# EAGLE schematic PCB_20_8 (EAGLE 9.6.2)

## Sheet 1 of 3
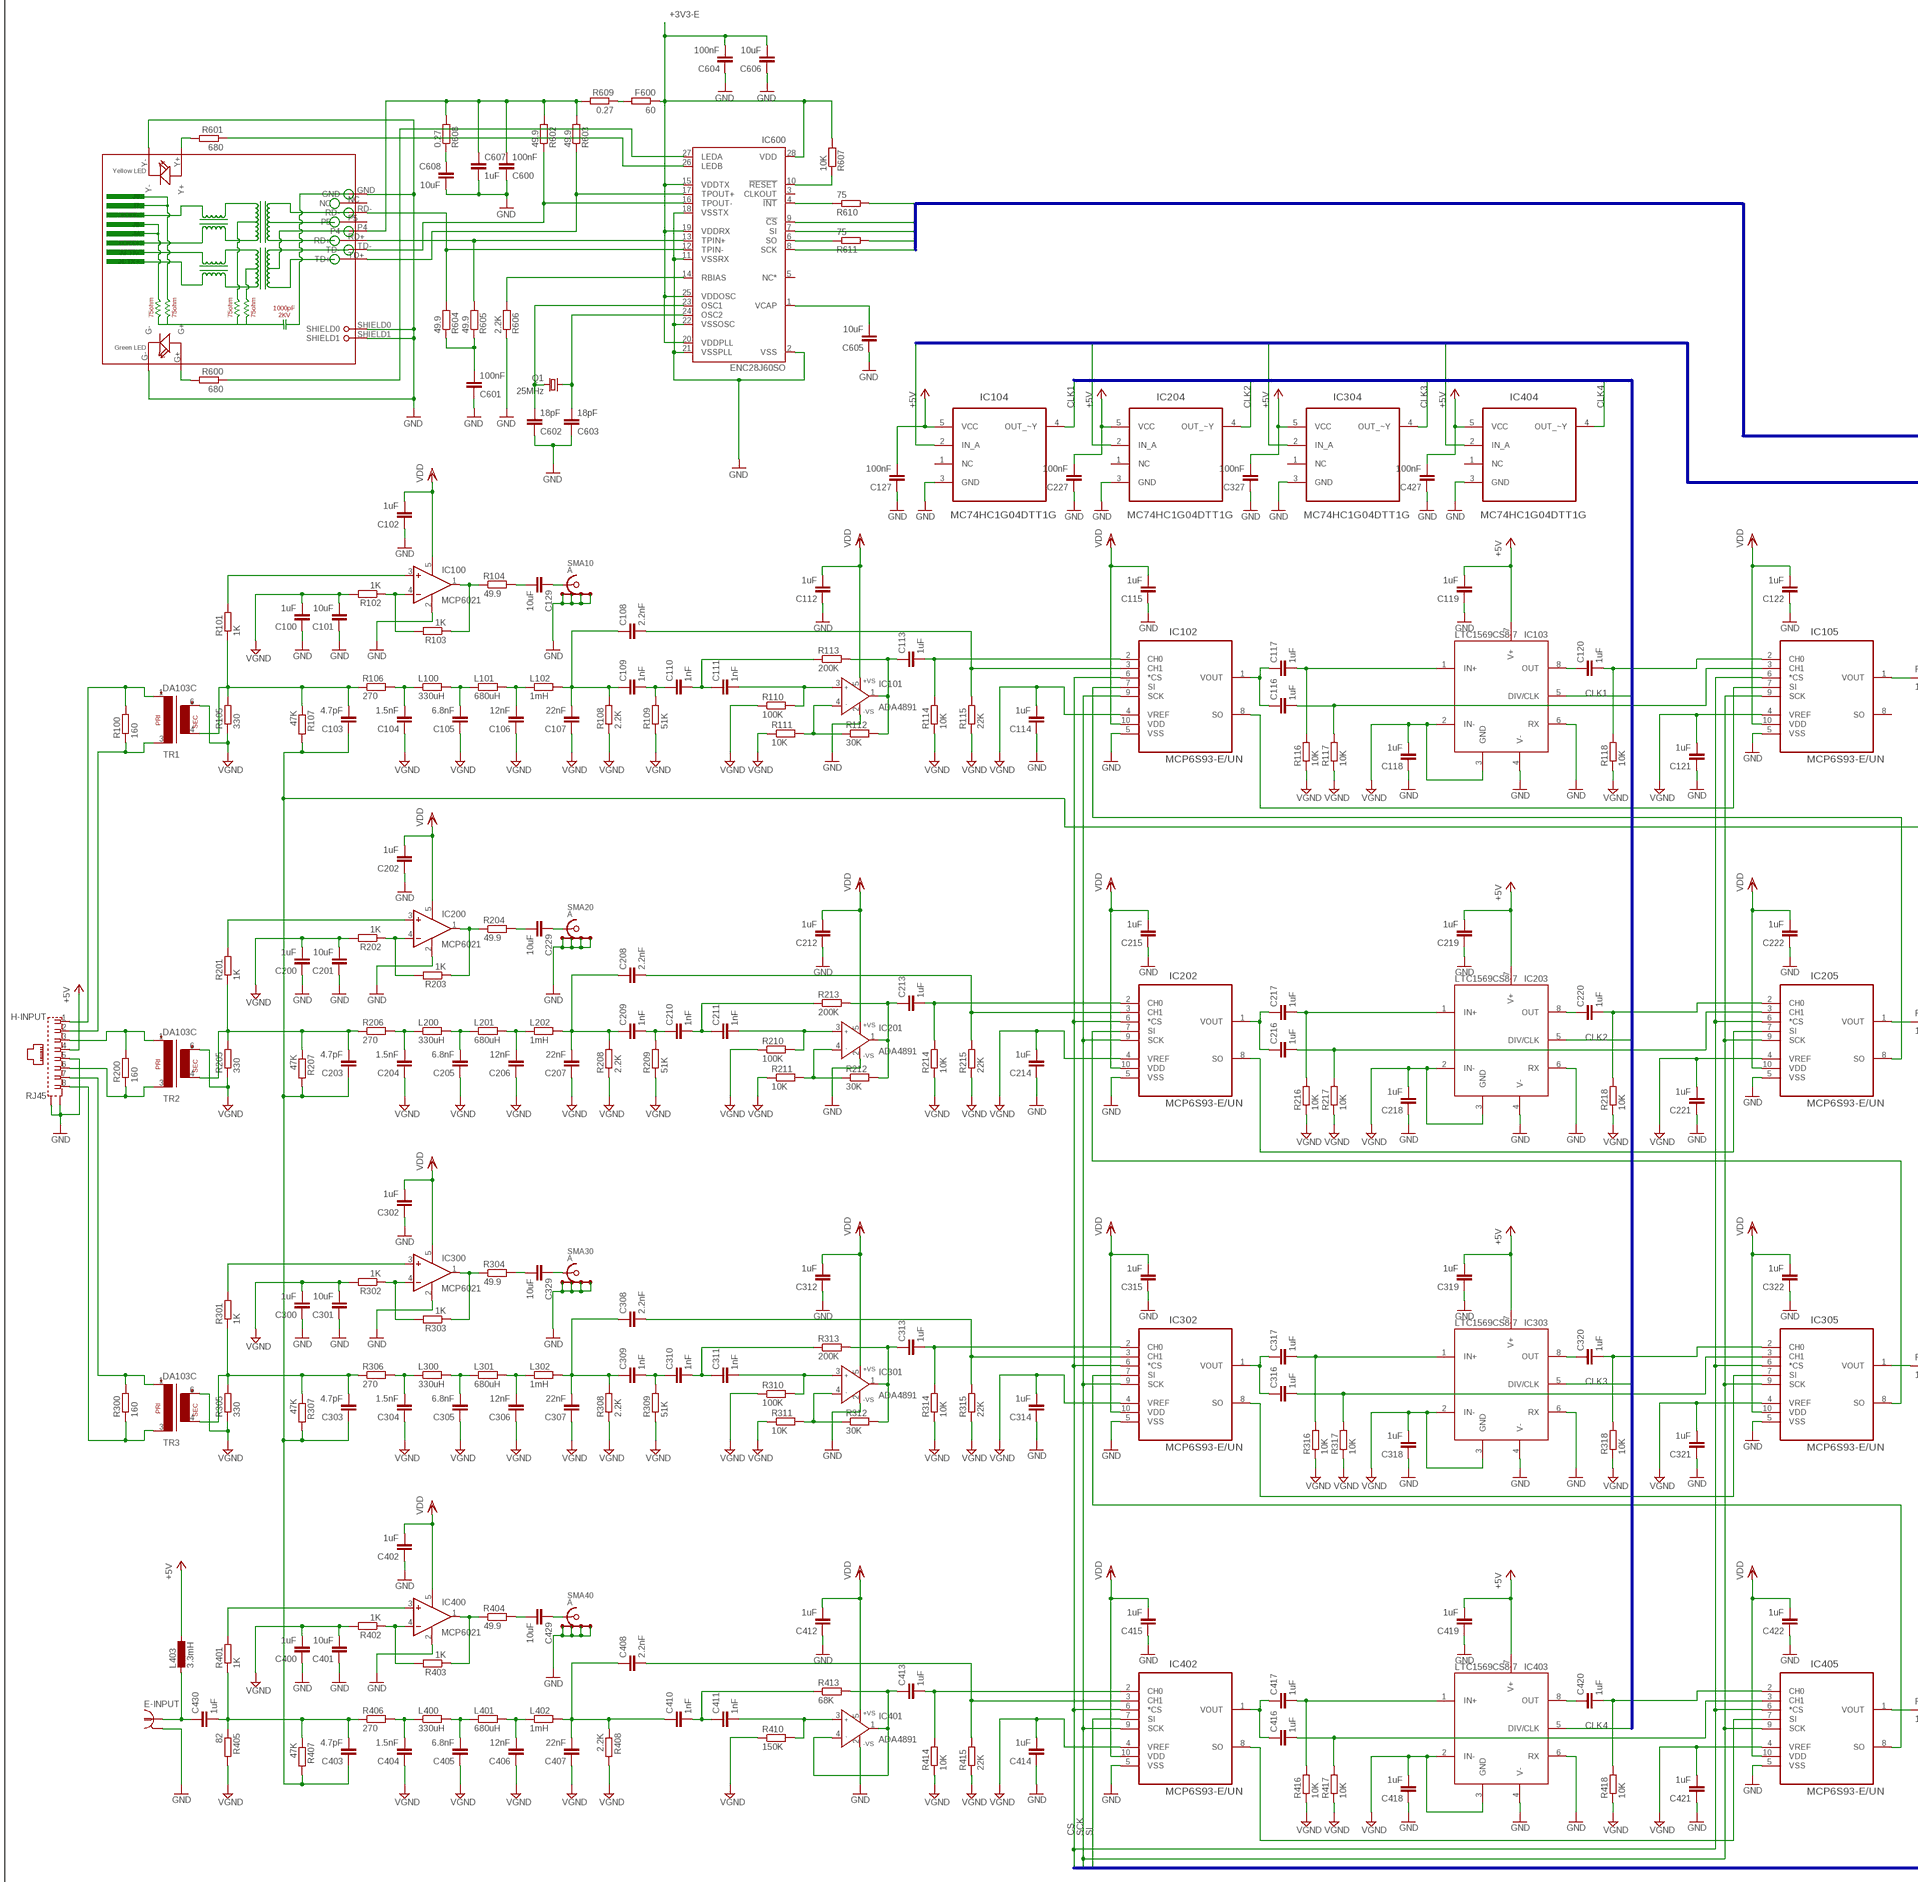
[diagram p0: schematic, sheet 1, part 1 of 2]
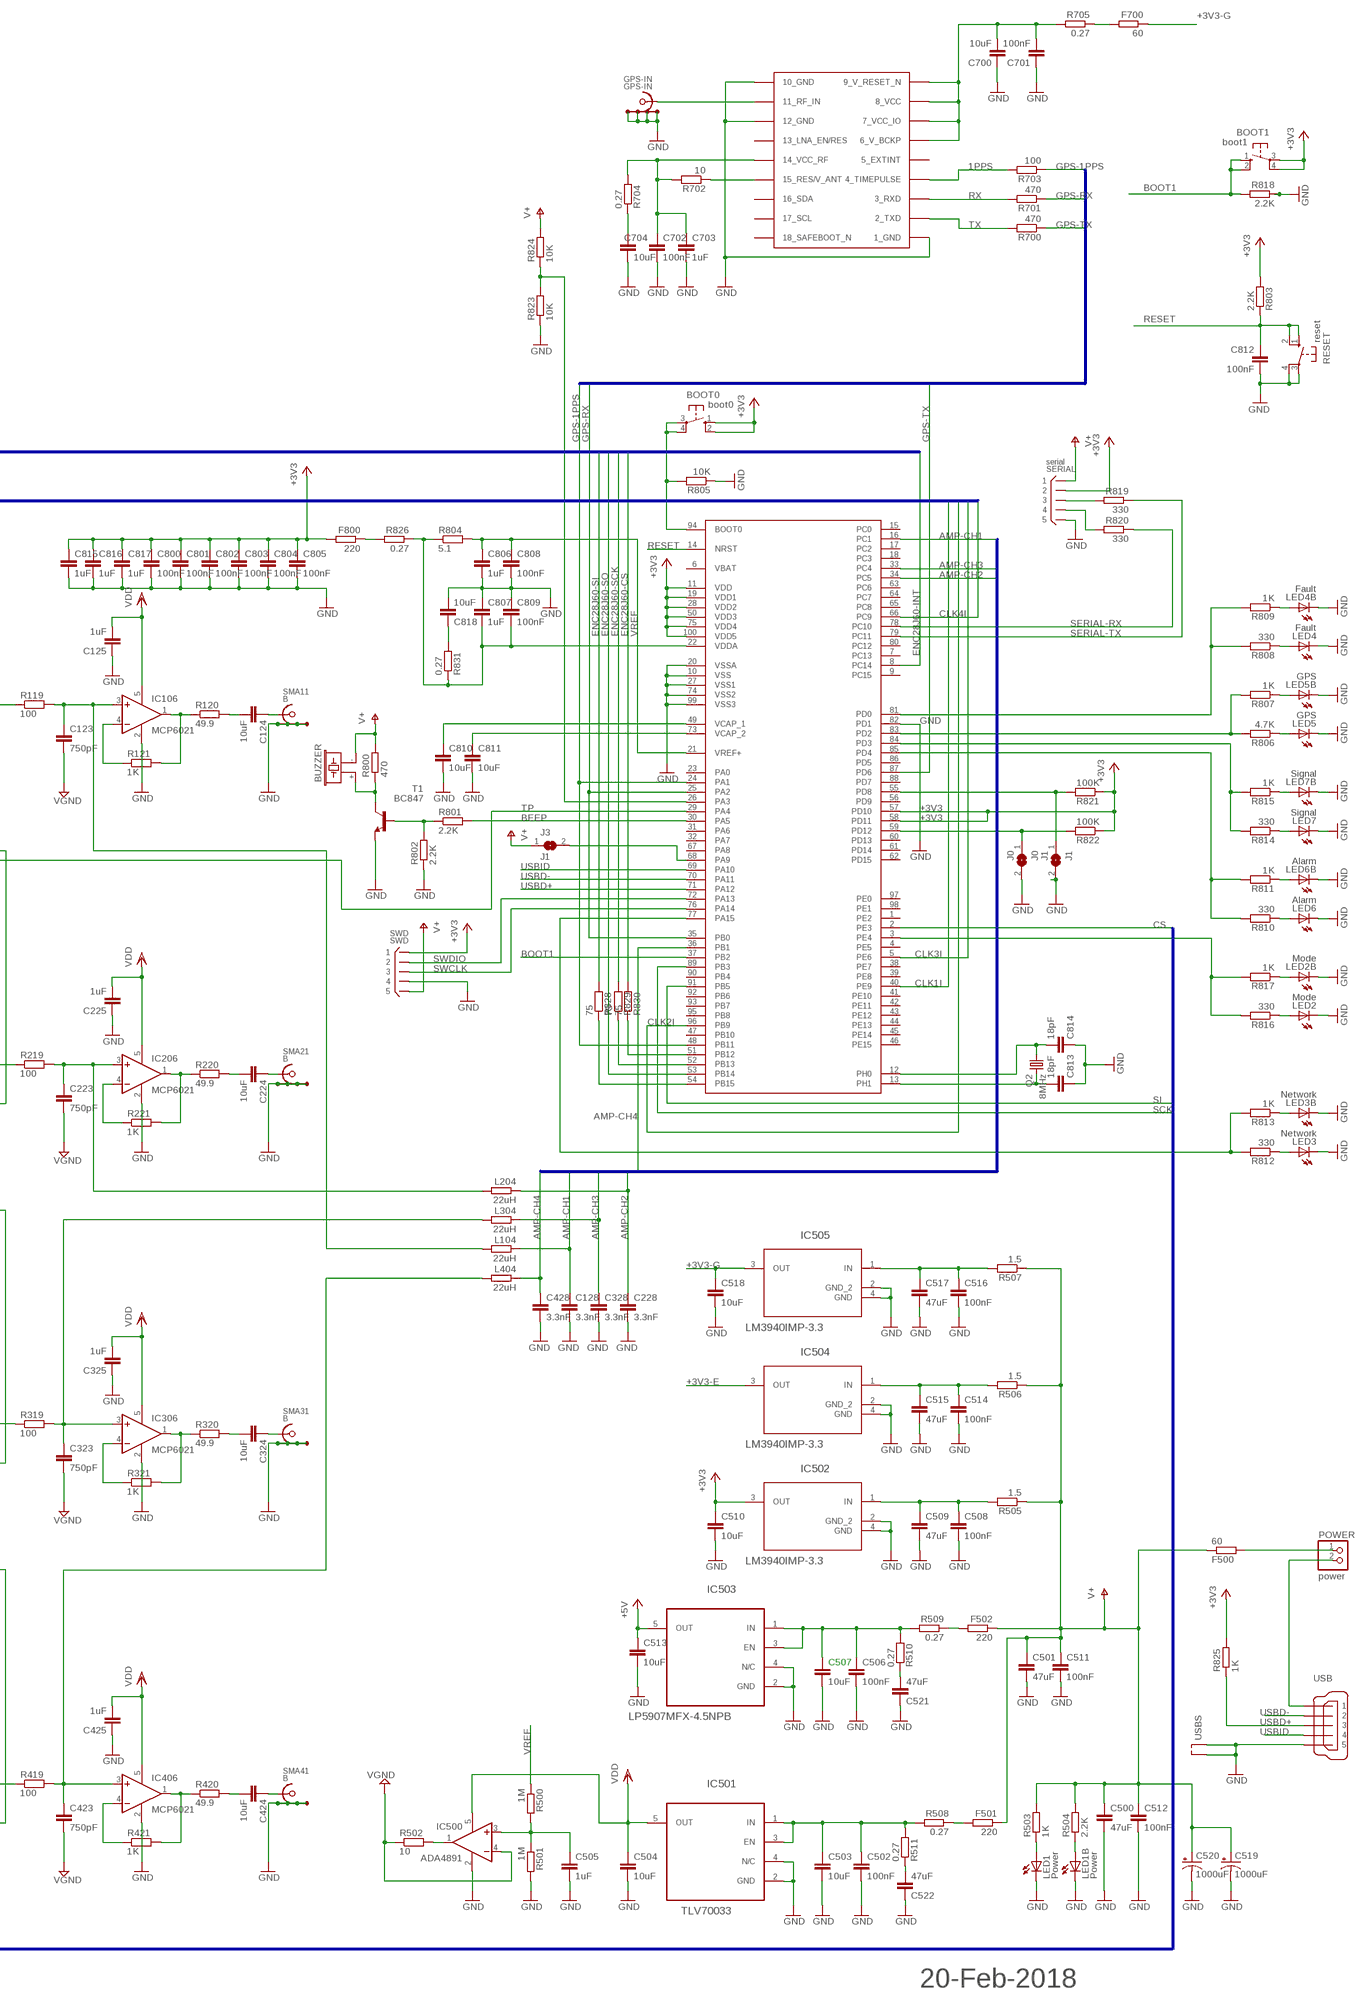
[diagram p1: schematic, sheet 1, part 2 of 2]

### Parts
BOOT0  boot0  10-XX  [B3F-10XX]
BOOT1  boot1  10-XX  [B3F-10XX]
BUZZER  F/CM12P  [F/CM12P]
C100  1uF  C-EUC0603  [C0603]
C101  10uF  C-EUC0805  [C0805]
C102  1uF  C-EUC0603  [C0603]
C103  4.7pF  C-EUC0603  [C0603]
C104  1.5nF  C-EUC0603  [C0603]
C105  6.8nF  C-EUC0603  [C0603]
C106  12nF  C-EUC0603  [C0603]
C107  22nF  C-EUC0603  [C0603]
C108  2.2nF  C-EUC0603  [C0603]
C109  1nF  C-EUC0603  [C0603]
C110  1nF  C-EUC0603  [C0603]
C111  1nF  C-EUC0603  [C0603]
C112  1uF  C-EUC0603  [C0603]
C113  1uF  C-EUC0603  [C0603]
C114  1uF  C-EUC0603  [C0603]
C115  1uF  C-EUC0603  [C0603]
C116  1uF  C-EUC0603  [C0603]
C117  1uF  C-EUC0603  [C0603]
C118  1uF  C-EUC0603  [C0603]
C119  1uF  C-EUC0603  [C0603]
C120  1uF  C-EUC0603  [C0603]
C121  1uF  C-EUC0603  [C0603]
C122  1uF  C-EUC0603  [C0603]
C123  750pF  C-EUC0603  [C0603]
C124  10uF  C-EUC0805  [C0805]
C125  1uF  C-EUC0603  [C0603]
C127  100nF  C-EUC0603  [C0603]
C128  3.3nF  C-EUC0603  [C0603]
C129  10uF  C-EUC0805  [C0805]
C200  1uF  C-EUC0603  [C0603]
C201  10uF  C-EUC0805  [C0805]
C202  1uF  C-EUC0603  [C0603]
C203  4.7pF  C-EUC0603  [C0603]
C204  1.5nF  C-EUC0603  [C0603]
C205  6.8nF  C-EUC0603  [C0603]
C206  12nF  C-EUC0603  [C0603]
C207  22nF  C-EUC0603  [C0603]
C208  2.2nF  C-EUC0603  [C0603]
C209  1nF  C-EUC0603  [C0603]
C210  1nF  C-EUC0603  [C0603]
C211  1nF  C-EUC0603  [C0603]
C212  1uF  C-EUC0603  [C0603]
C213  1uF  C-EUC0603  [C0603]
C214  1uF  C-EUC0603  [C0603]
C215  1uF  C-EUC0603  [C0603]
C216  1uF  C-EUC0603  [C0603]
C217  1uF  C-EUC0603  [C0603]
C218  1uF  C-EUC0603  [C0603]
C219  1uF  C-EUC0603  [C0603]
C220  1uF  C-EUC0603  [C0603]
C221  1uF  C-EUC0603  [C0603]
C222  1uF  C-EUC0603  [C0603]
C223  750pF  C-EUC0603  [C0603]
C224  10uF  C-EUC0805  [C0805]
C225  1uF  C-EUC0603  [C0603]
C227  100nF  C-EUC0603  [C0603]
C228  3.3nF  C-EUC0603  [C0603]
C229  10uF  C-EUC0805  [C0805]
C300  1uF  C-EUC0603  [C0603]
C301  10uF  C-EUC0805  [C0805]
C302  1uF  C-EUC0603  [C0603]
C303  4.7pF  C-EUC0603  [C0603]
C304  1.5nF  C-EUC0603  [C0603]
C305  6.8nF  C-EUC0603  [C0603]
C306  12nF  C-EUC0603  [C0603]
C307  22nF  C-EUC0603  [C0603]
C308  2.2nF  C-EUC0603  [C0603]
C309  1nF  C-EUC0603  [C0603]
C310  1nF  C-EUC0603  [C0603]
C311  1nF  C-EUC0603  [C0603]
C312  1uF  C-EUC0603  [C0603]
C313  1uF  C-EUC0603  [C0603]
C314  1uF  C-EUC0603  [C0603]
C315  1uF  C-EUC0603  [C0603]
C316  1uF  C-EUC0603  [C0603]
C317  1uF  C-EUC0603  [C0603]
C318  1uF  C-EUC0603  [C0603]
C319  1uF  C-EUC0603  [C0603]
C320  1uF  C-EUC0603  [C0603]
C321  1uF  C-EUC0603  [C0603]
C322  1uF  C-EUC0603  [C0603]
C323  750pF  C-EUC0603  [C0603]
C324  10uF  C-EUC0805  [C0805]
C325  1uF  C-EUC0603  [C0603]
C327  100nF  C-EUC0603  [C0603]
C328  3.3nF  C-EUC0603  [C0603]
C329  10uF  C-EUC0805  [C0805]
C400  1uF  C-EUC0603  [C0603]
C401  10uF  C-EUC0805  [C0805]
C402  1uF  C-EUC0603  [C0603]
C403  4.7pF  C-EUC0603  [C0603]
C404  1.5nF  C-EUC0603  [C0603]
C405  6.8nF  C-EUC0603  [C0603]
C406  12nF  C-EUC0603  [C0603]
C407  22nF  C-EUC0603  [C0603]
C408  2.2nF  C-EUC0603  [C0603]
C410  1nF  C-EUC0603  [C0603]
C411  1nF  C-EUC0603  [C0603]
C412  1uF  C-EUC0603  [C0603]
C413  1uF  C-EUC0603  [C0603]
C414  1uF  C-EUC0603  [C0603]
C415  1uF  C-EUC0603  [C0603]
C416  1uF  C-EUC0603  [C0603]
C417  1uF  C-EUC0603  [C0603]
C418  1uF  C-EUC0603  [C0603]
C419  1uF  C-EUC0603  [C0603]
C420  1uF  C-EUC0603  [C0603]
C421  1uF  C-EUC0603  [C0603]
C422  1uF  C-EUC0603  [C0603]
C423  750pF  C-EUC0603  [C0603]
C424  10uF  C-EUC0805  [C0805]
C425  1uF  C-EUC0603  [C0603]
C427  100nF  C-EUC0603  [C0603]
C428  3.3nF  C-EUC0603  [C0603]
C429  10uF  C-EUC0805  [C0805]
C430  1uF  C-EUC0603  [C0603]
C500  47uF  C-EUC1210  [C1210]
C501  47uF  C-EUC1210  [C1210]
C502  100nF  C-EUC0603  [C0603]
C503  10uF  C-EUC0805  [C0805]
C504  10uF  C-EUC0805  [C0805]
C505  1uF  C-EUC0603  [C0603]
C506  100nF  C-EUC0603  [C0603]
C507  10uF  C-EUC0805  [C0805]
C508  100nF  C-EUC0603  [C0603]
C509  47uF  C-EUC1210  [C1210]
C510  10uF  C-EUC0805  [C0805]
C511  100nF  C-EUC0603  [C0603]
C512  100nF  C-EUC0603  [C0603]
C513  10uF  C-EUC0805  [C0805]
C514  100nF  C-EUC0603  [C0603]
C515  47uF  C-EUC1210  [C1210]
C516  100nF  C-EUC0603  [C0603]
C517  47uF  C-EUC1210  [C1210]
C518  10uF  C-EUC0805  [C0805]
C519  1000uF  CPOL-USE5-10.5  [E5-10,5]
C520  1000uF  CPOL-USE5-10.5  [E5-10,5]
C521  47uF  C-EUC1210  [C1210]
C522  47uF  C-EUC1210  [C1210]
C600  100nF  C-EUC0603  [C0603]
C601  100nF  C-EUC0603  [C0603]
C602  18pF  C-EUC0603  [C0603]
C603  18pF  C-EUC0603  [C0603]
C604  100nF  C-EUC0603  [C0603]
C605  10uF  C-EUC0805  [C0805]
C606  10uF  C-EUC0805  [C0805]
C607  1uF  C-EUC0603  [C0603]
C608  10uF  C-EUC0805  [C0805]
C700  10uF  C-EUC0805  [C0805]
C701  100nF  C-EUC0603  [C0603]
C702  100nF  C-EUC0603  [C0603]
C703  1uF  C-EUC0603  [C0603]
C704  10uF  C-EUC0805  [C0805]
C800  100nF  C-EUC0603  [C0603]
C801  100nF  C-EUC0603  [C0603]
C802  100nF  C-EUC0603  [C0603]
C803  100nF  C-EUC0603  [C0603]
C804  100nF  C-EUC0603  [C0603]
C805  100nF  C-EUC0603  [C0603]
C806  1uF  C-EUC0603  [C0603]
C807  1uF  C-EUC0603  [C0603]
C808  100nF  C-EUC0603  [C0603]
C809  100nF  C-EUC0603  [C0603]
C810  10uF  C-EUC0805  [C0805]
C811  10uF  C-EUC0805  [C0805]
C812  100nF  C-EUC0603  [C0603]
C813  18pF  C-EUC0603  [C0603]
C814  18pF  C-EUC0603  [C0603]
C815  1uF  C-EUC0603  [C0603]
C816  1uF  C-EUC0603  [C0603]
C817  1uF  C-EUC0603  [C0603]
C818  10uF  C-EUC0805  [C0805]
E-INPUT  R141426  [R141426]
F500  60  R-EU_R0805  [R0805]
F501  220  R-EU_R0805  [R0805]
F502  220  R-EU_R0805  [R0805]
F600  60  R-EU_R0805  [R0805]
F700  60  R-EU_R0805  [R0805]
F800  220  R-EU_R0805  [R0805]
GPS-IN  GPS-IN  XS-4S-LEMO00V  [XLEMO02N]
H-INPUT  RJ45  556591-1  [556591-1]
IC100  MCP6021  OPA344N-SOT23  [SOT23-5]
IC101  ADA4891  AD8614RJ  [SOT23-5]
IC102  MCP6S93-E/UN  [SOP50P490X110-10N]
IC103  LTC1569CS8-7  LTC1569-7  [SOIC8]
IC104  MC74HC1G04DTT1G  [SOT95P275X110-5N]
IC105  MCP6S93-E/UN  [SOP50P490X110-10N]
IC106  MCP6021  OPA344N-SOT23  [SOT23-5]
IC200  MCP6021  OPA344N-SOT23  [SOT23-5]
IC201  ADA4891  AD8614RJ  [SOT23-5]
IC202  MCP6S93-E/UN  [SOP50P490X110-10N]
IC203  LTC1569CS8-7  LTC1569-7  [SOIC8]
IC204  MC74HC1G04DTT1G  [SOT95P275X110-5N]
IC205  MCP6S93-E/UN  [SOP50P490X110-10N]
IC206  MCP6021  OPA344N-SOT23  [SOT23-5]
IC300  MCP6021  OPA344N-SOT23  [SOT23-5]
IC301  ADA4891  AD8614RJ  [SOT23-5]
IC302  MCP6S93-E/UN  [SOP50P490X110-10N]
IC303  LTC1569CS8-7  LTC1569-7  [SOIC8]
IC304  MC74HC1G04DTT1G  [SOT95P275X110-5N]
IC305  MCP6S93-E/UN  [SOP50P490X110-10N]
IC306  MCP6021  OPA344N-SOT23  [SOT23-5]
IC400  MCP6021  OPA344N-SOT23  [SOT23-5]
IC401  ADA4891  AD8614RJ  [SOT23-5]
IC402  MCP6S93-E/UN  [SOP50P490X110-10N]
IC403  LTC1569CS8-7  LTC1569-7  [SOIC8]
IC404  MC74HC1G04DTT1G  [SOT95P275X110-5N]
IC405  MCP6S93-E/UN  [SOP50P490X110-10N]
IC406  MCP6021  OPA344N-SOT23  [SOT23-5]
IC500  ADA4891  OPA344N-SOT23  [SOT23-5]
IC501  TLV70033  TLV70033DDCT  [SOT95P280X110-5N]
IC502  LM3940IMP-3.3  [SOT230P696X180-4N]
IC503  LP5907MFX-4.5NPB  TLV70033DDCT  [SOT95P280X110-5N]
IC504  LM3940IMP-3.3  [SOT230P696X180-4N]
IC505  LM3940IMP-3.3  [SOT230P696X180-4N]
IC600  ENC28J60SO  [SO28W]
IC800  STM32D40X  STM32F40XSTM32D40X  [LQFP100]
J0  J0  SJ  [SJ]
J1  J1  SJ  [SJ]
J3  J1  SJ  [SJ]
L100  330uH  R-EU_R1210  [R1210]
L101  680uH  R-EU_R1210  [R1210]
L102  1mH  R-EU_R1210  [R1210]
L104  22uH  R-EU_R1210  [R1210]
L200  330uH  R-EU_R1210  [R1210]
L201  680uH  R-EU_R1210  [R1210]
L202  1mH  R-EU_R1210  [R1210]
L204  22uH  R-EU_R1210  [R1210]
L300  330uH  R-EU_R1210  [R1210]
L301  680uH  R-EU_R1210  [R1210]
L302  1mH  R-EU_R1210  [R1210]
L304  22uH  R-EU_R1210  [R1210]
L400  330uH  R-EU_R1210  [R1210]
L401  680uH  R-EU_R1210  [R1210]
L402  1mH  R-EU_R1210  [R1210]
L403  3.3mH  L-EU6000-XXX-RC  [6000-XXXX-RC]
L404  22uH  R-EU_R1210  [R1210]
LED1  Power  LED3MM  [LED3MM]
LED1B  Power  LEDCHIP-LED0805  [CHIP-LED0805]
LED2  Mode  LED3MM  [LED3MM]
LED2B  Mode  LEDCHIP-LED0805  [CHIP-LED0805]
LED3  Network  LED3MM  [LED3MM]
LED3B  Network  LEDCHIP-LED0805  [CHIP-LED0805]
LED4  Fault  LED3MM  [LED3MM]
LED4B  Fault  LEDCHIP-LED0805  [CHIP-LED0805]
LED5  GPS  LED3MM  [LED3MM]
LED5B  GPS  LEDCHIP-LED0805  [CHIP-LED0805]
LED6  Alarm  LED3MM  [LED3MM]
LED6B  Alarm  LEDCHIP-LED0805  [CHIP-LED0805]
LED7  Signal  LED3MM  [LED3MM]
LED7B  Signal  LEDCHIP-LED0805  [CHIP-LED0805]
POWER  power  PINHD-1X2  [1X02]
Q1  25MHz  CRYSTALHC49U-V  [HC49U-V]
Q2  8MHz  CRYSTALHC49U-V  [HC49U-V]
R100  160  R-EU_R0603  [R0603]
R101  1K  R-EU_R0603  [R0603]
R102  1K  R-EU_R0603  [R0603]
R103  1K  R-EU_R0603  [R0603]
R104  49.9  R-EU_R0603  [R0603]
R105  330  R-EU_R0603  [R0603]
R106  270  R-EU_R0603  [R0603]
R107  47K  R-EU_R0603  [R0603]
R108  2.2K  R-EU_R0603  [R0603]
R109  51K  R-EU_R0603  [R0603]
R110  100K  R-EU_R0603  [R0603]
R111  10K  R-EU_R0603  [R0603]
R112  30K  R-EU_R0603  [R0603]
R113  200K  R-EU_R0603  [R0603]
R114  10K  R-EU_R0603  [R0603]
R115  22K  R-EU_R0603  [R0603]
R116  10K  R-EU_R0603  [R0603]
R117  10K  R-EU_R0603  [R0603]
R118  10K  R-EU_R0603  [R0603]
R119  100  R-EU_R0603  [R0603]
R120  49.9  R-EU_R0603  [R0603]
R121  1K  R-EU_R0603  [R0603]
R200  160  R-EU_R0603  [R0603]
R201  1K  R-EU_R0603  [R0603]
R202  1K  R-EU_R0603  [R0603]
R203  1K  R-EU_R0603  [R0603]
R204  49.9  R-EU_R0603  [R0603]
R205  330  R-EU_R0603  [R0603]
R206  270  R-EU_R0603  [R0603]
R207  47K  R-EU_R0603  [R0603]
R208  2.2K  R-EU_R0603  [R0603]
R209  51K  R-EU_R0603  [R0603]
R210  100K  R-EU_R0603  [R0603]
R211  10K  R-EU_R0603  [R0603]
R212  30K  R-EU_R0603  [R0603]
R213  200K  R-EU_R0603  [R0603]
R214  10K  R-EU_R0603  [R0603]
R215  22K  R-EU_R0603  [R0603]
R216  10K  R-EU_R0603  [R0603]
R217  10K  R-EU_R0603  [R0603]
R218  10K  R-EU_R0603  [R0603]
R219  100  R-EU_R0603  [R0603]
R220  49.9  R-EU_R0603  [R0603]
R221  1K  R-EU_R0603  [R0603]
R300  160  R-EU_R0603  [R0603]
R301  1K  R-EU_R0603  [R0603]
R302  1K  R-EU_R0603  [R0603]
R303  1K  R-EU_R0603  [R0603]
R304  49.9  R-EU_R0603  [R0603]
R305  330  R-EU_R0603  [R0603]
R306  270  R-EU_R0603  [R0603]
R307  47K  R-EU_R0603  [R0603]
R308  2.2K  R-EU_R0603  [R0603]
R309  51K  R-EU_R0603  [R0603]
R310  100K  R-EU_R0603  [R0603]
R311  10K  R-EU_R0603  [R0603]
R312  30K  R-EU_R0603  [R0603]
R313  200K  R-EU_R0603  [R0603]
R314  10K  R-EU_R0603  [R0603]
R315  22K  R-EU_R0603  [R0603]
R316  10K  R-EU_R0603  [R0603]
R317  10K  R-EU_R0603  [R0603]
R318  10K  R-EU_R0603  [R0603]
R319  100  R-EU_R0603  [R0603]
R320  49.9  R-EU_R0603  [R0603]
R321  1K  R-EU_R0603  [R0603]
R401  1K  R-EU_R0603  [R0603]
R402  1K  R-EU_R0603  [R0603]
R403  1K  R-EU_R0603  [R0603]
R404  49.9  R-EU_R0603  [R0603]
R405  82  R-EU_R0603  [R0603]
R406  270  R-EU_R0603  [R0603]
R407  47K  R-EU_R0603  [R0603]
R408  2.2K  R-EU_R0603  [R0603]
R410  150K  R-EU_R0603  [R0603]
R413  68K  R-EU_R0603  [R0603]
R414  10K  R-EU_R0603  [R0603]
R415  22K  R-EU_R0603  [R0603]
R416  10K  R-EU_R0603  [R0603]
R417  10K  R-EU_R0603  [R0603]
R418  10K  R-EU_R0603  [R0603]
R419  100  R-EU_R0603  [R0603]
R420  49.9  R-EU_R0603  [R0603]
R421  1K  R-EU_R0603  [R0603]
R500  1M  R-EU_R0603  [R0603]
R501  1M  R-EU_R0603  [R0603]
R502  10  R-EU_R0603  [R0603]
R503  1K  R-EU_R0603  [R0603]
R504  2.2K  R-EU_R0603  [R0603]
R505  1.5  R-EU_R2512  [R2512]
R506  1.5  R-EU_R2512  [R2512]
R507  1.5  R-EU_R2512  [R2512]
R508  0.27  R-EU_R0603  [R0603]
R509  0.27  R-EU_R0603  [R0603]
R510  0.27  R-EU_R0603  [R0603]
R511  0.27  R-EU_R0603  [R0603]
R600  680  R-EU_R0603  [R0603]
R601  680  R-EU_R0603  [R0603]
R602  49.9  R-EU_R0603  [R0603]
R603  49.9  R-EU_R0603  [R0603]
R604  49.9  R-EU_R0603  [R0603]
R605  49.9  R-EU_R0603  [R0603]
R606  2.2K  R-EU_R0603  [R0603]
R607  10K  R-EU_R0603  [R0603]
R608  0.27  R-EU_R0603  [R0603]
R609  0.27  R-EU_R0603  [R0603]
R610  75  R-EU_R0603  [R0603]
R611  75  R-EU_R0603  [R0603]
R700  470  R-EU_R0603  [R0603]
R701  470  R-EU_R0603  [R0603]
R702  10  R-EU_R0603  [R0603]
R703  100  R-EU_R0603  [R0603]
R704  0.27  R-EU_R0603  [R0603]
R705  0.27  R-EU_R0603  [R0603]
R800  470  R-EU_R0603  [R0603]
R801  2.2K  R-EU_R0603  [R0603]
R802  2.2K  R-EU_R0603  [R0603]
R803  2.2K  R-EU_R0603  [R0603]
R804  5.1  R-EU_R0603  [R0603]
R805  10K  R-EU_R0603  [R0603]
R806  4.7K  R-EU_R0603  [R0603]
R807  1K  R-EU_R0603  [R0603]
R808  330  R-EU_R0603  [R0603]
R809  1K  R-EU_R0603  [R0603]
R810  330  R-EU_R0603  [R0603]
R811  1K  R-EU_R0603  [R0603]
R812  330  R-EU_R0603  [R0603]
R813  1K  R-EU_R0603  [R0603]
R814  330  R-EU_R0603  [R0603]
R815  1K  R-EU_R0603  [R0603]
R816  330  R-EU_R0603  [R0603]
R817  1K  R-EU_R0603  [R0603]
R818  2.2K  R-EU_R0603  [R0603]
R819  330  R-EU_R0603  [R0603]
R820  330  R-EU_R0603  [R0603]
R821  100K  R-EU_R0603  [R0603]
R822  100K  R-EU_R0603  [R0603]
R823  10K  R-EU_R0603  [R0603]
R824  10K  R-EU_R0603  [R0603]
R825  1K  R-EU_R0603  [R0603]
R826  0.27  R-EU_R0603  [R0603]
R828  75  R-EU_R0603  [R0603]
R829  75  R-EU_R0603  [R0603]
R830  75  R-EU_R0603  [R0603]
R831  0.27  R-EU_R0603  [R0603]
RESET  reset  10-XX  [B3F-10XX]
RJ1  HR911105A  [HR911105A]
SERIAL  serial  X05N  [X05N-SIL]
SMA10  A  XS-4S-LEMO00V  [XLEMO02N]
SMA11  B  XS-4S-LEMO00V  [XLEMO02N]
SMA20  A  XS-4S-LEMO00V  [XLEMO02N]
SMA21  B  XS-4S-LEMO00V  [XLEMO02N]
SMA30  A  XS-4S-LEMO00V  [XLEMO02N]
SMA31  B  XS-4S-LEMO00V  [XLEMO02N]
SMA40  A  XS-4S-LEMO00V  [XLEMO02N]
SMA41  B  XS-4S-LEMO00V  [XLEMO02N]
SWD  SWD  X05N  [X05N-SIL]
T1  BC847  BC847SMD  [SOT23]
TR1  DA103C  78601  [786-4]
TR2  DA103C  78601  [786-4]
TR3  DA103C  78601  [786-4]
U$1  MAX-M8  [MAX-M8]
USB  MINI-USB_SHIELD5P2-32005-601  [32005-601]

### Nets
1PPS: R703.2 U$1.4_TIMEPULSE
+3V3: BOOT0.1(S) BOOT0.2(S1) BOOT1.3(P) BOOT1.4(P1) C510.1 C800.1 C801.1 C802.1 C803.1 C804.1 C805.1 C815.1 C816.1 C817.1 F800.2 IC502.3(OUT) IC800.11(VDD) IC800.19(VDD1) IC800.28(VDD2) IC800.50(VDD3) IC800.57(PD10) IC800.58(PD11) IC800.75(VDD4) IC800.100(VDD5) R803.2 R821.1 R822.1 R825.2 SERIAL.2 SWD.1
+3V3-E: C604.2 C606.2 F600.1 IC504.3(OUT) IC600.15(VDDTX) IC600.19(VDDRX) IC600.20(VDDPLL) IC600.25(VDDOSC) IC600.28(VDD) R607.2
+3V3-G: C518.1 F700.1 IC505.3(OUT)
+5V: C119.2 C127.2 C219.2 C227.2 C319.2 C327.2 C419.2 C427.2 C513.1 H-INPUT.4 IC103.7(V+) IC104.5(VCC) IC203.7(V+) IC204.5(VCC) IC303.7(V+) IC304.5(VCC) IC403.7(V+) IC404.5(VCC) IC503.5(OUT) L403.1
AGND: C100.2 C101.2 C104.1 C105.1 C106.1 C107.1 C114.2 C118.2 C121.2 C123.2 C200.2 C201.2 C204.1 C205.1 C206.1 C207.1 C214.2 C218.2 C221.2 C223.2 C300.2 C301.2 C304.1 C305.1 C306.1 C307.1 C314.2 C318.2 C321.2 C323.2 C400.2 C401.2 C404.1 C405.1 C406.1 C407.1 C414.2 C418.2 C421.2 C423.2 IC102.4(VREF) IC103.2(IN-) IC103.3(GND) IC105.4(VREF) IC202.4(VREF) IC203.2(IN-) IC203.3(GND) IC205.4(VREF) IC302.4(VREF) IC303.2(IN-) IC303.3(GND) IC305.4(VREF) IC402.4(VREF) IC403.2(IN-) IC403.3(GND) IC405.4(VREF) IC500.4(-IN) R102.2 R105.1 R108.1 R109.1 R110.1 R111.1 R114.1 R115.1 R116.1 R117.1 R118.1 R202.2 R205.1 R208.1 R209.1 R210.1 R211.1 R214.1 R215.1 R216.1 R217.1 R218.1 R302.2 R305.1 R308.1 R309.1 R310.1 R311.1 R314.1 R315.1 R316.1 R317.1 R318.1 R402.2 R405.2 R408.2 R410.1 R414.1 R415.1 R416.1 R417.1 R418.1 R502.1 TR1.6(S1) TR2.6(S1) TR3.6(S1) ; supply symbol labelled VGND
AMP-CH1: C128.1 IC800.16(PC1) L104.1
AMP-CH2: C228.1 IC800.34(PC5) L204.1
AMP-CH3: C328.1 IC800.33(PC4) L304.1
AMP-CH4: C428.1 IC800.36(PB1) L404.1
BEEP: IC800.30(PA5) R801.2
BNC2A: C123.1 IC106.3(+IN) L104.2 R119.2
BNC2B: C223.1 IC206.3(+IN) L204.2 R219.2
BNC2D: C423.1 IC406.3(+IN) L404.2 R419.2
BOOT1: BOOT1.1(S) BOOT1.2(S1) IC800.37(PB2) R818.2
C106: C103.2 R101.1 R105.2 R106.1 R107.1 TR1.4(S2)
CLK1: IC103.5(DIV/CLK) IC104.4(OUT_~Y)
CLK1I: IC104.2(IN_A) IC800.40(PE9)
CLK2: IC203.5(DIV/CLK) IC204.4(OUT_~Y)
CLK2I: IC204.2(IN_A) IC800.96(PB9)
CLK3: IC303.5(DIV/CLK) IC304.4(OUT_~Y)
CLK3I: IC304.2(IN_A) IC800.5(PE6)
CLK4: IC403.5(DIV/CLK) IC404.4(OUT_~Y)
CLK4I: IC404.2(IN_A) IC800.66(PC9)
CS: IC102.6(*CS) IC105.6(*CS) IC202.6(*CS) IC205.6(*CS) IC302.6(*CS) IC305.6(*CS) IC402.6(*CS) IC405.6(*CS) IC800.2(PE3)
ENC28J60-CS: IC600.9(!CS) R830.2
ENC28J60-INT: IC800.8(PC14) R610.2
ENC28J60-INT-A: IC600.4(!INT) R610.1
ENC28J60-SCK: IC600.8(SCK) R829.2
ENC28J60-SI: IC600.7(SI) R828.2
ENC28J60-SO: IC800.53(PB14) R611.2
ENC28J60-SO-A: IC600.6(SO) R611.1
GND: C100.1 C101.1 C102.1 C112.1 C114.1 C115.1 C118.1 C119.1 C121.1 C122.1 C125.1 C127.1 C128.2 C200.1 C201.1 C202.1 C212.1 C214.1 C215.1 C218.1 C219.1 C221.1 C222.1 C225.1 C227.1 C228.2 C300.1 C301.1 C302.1 C312.1 C314.1 C315.1 C318.1 C319.1 C321.1 C322.1 C325.1 C327.1 C328.2 C400.1 C401.1 C402.1 C412.1 C414.1 C415.1 C418.1 C419.1 C421.1 C422.1 C425.1 C427.1 C428.2 C500.2 C501.2 C502.2 C503.2 C504.2 C505.2 C506.2 C507.2 C508.2 C509.2 C510.2 C511.2 C512.2 C513.2 C514.2 C515.2 C516.2 C517.2 C518.2 C519.- C520.- C521.1 C522.1 C600.1 C601.1 C602.1 C603.1 C604.1 C605.1 C606.1 C607.2 C608.2 C700.1 C701.1 C702.2 C703.2 C704.2 C800.2 C801.2 C802.2 C803.2 C804.2 C805.2 C806.2 C807.1 C808.2 C809.1 C810.2 C811.2 C812.2 C813.1 C814.1 C815.2 C816.2 C817.2 C818.2 E-INPUT.2(GND) GPS-IN.GND@1(GND) GPS-IN.GND@2(GND) GPS-IN.GND@3(GND) GPS-IN.GND@4(GND) H-INPUT.5 H-INPUT.G1(S1) H-INPUT.G2(S2) IC100.2(V-) IC101.2(-VS) IC102.5(VSS) IC103.4(V-) IC103.6(RX) IC104.3(GND) IC105.5(VSS) IC106.2(V-) IC200.2(V-) IC201.2(-VS) IC202.5(VSS) IC203.4(V-) IC203.6(RX) IC204.3(GND) IC205.5(VSS) IC206.2(V-) IC300.2(V-) IC301.2(-VS) IC302.5(VSS) IC303.4(V-) IC303.6(RX) IC304.3(GND) IC305.5(VSS) IC306.2(V-) IC400.2(V-) IC401.2(-VS) IC402.5(VSS) IC403.4(V-) IC403.6(RX) IC404.3(GND) IC405.5(VSS) IC406.2(V-) IC500.2(V-) IC501.2(GND) IC501.4(N/C) IC502.2(GND_2) IC502.4(GND) IC503.2(GND) IC503.4(N/C) IC504.2(GND_2) IC504.4(GND) IC505.2(GND_2) IC505.4(GND) IC600.2(VSS) IC600.11(VSSRX) IC600.18(VSSTX) IC600.21(VSSPLL) IC600.22(VSSOSC) IC800.10(VSS) IC800.20(VSSA) IC800.27(VSS1) IC800.74(VSS2) IC800.82(PD1) IC800.99(VSS3) J0.2 J1.2 LED1.K(C) LED1B.C LED2.K(C) LED2B.C LED3.K(C) LED3B.C LED4.K(C) LED4B.C LED5.K(C) LED5B.C LED6.K(C) LED6B.C LED7.K(C) LED7B.C R501.2 R606.1 R802.1 R805.1 R818.1 R823.1 RESET.3(P) RESET.4(P1) RJ1.G- RJ1.GND RJ1.SHIELD0 RJ1.SHIELD1 RJ1.Y- SERIAL.5 SMA10.GND@1(GND) SMA10.GND@2(GND) SMA10.GND@3(GND) SMA10.GND@4(GND) SMA11.GND@1(GND) SMA11.GND@2(GND) SMA11.GND@3(GND) SMA11.GND@4(GND) SMA20.GND@1(GND) SMA20.GND@2(GND) SMA20.GND@3(GND) SMA20.GND@4(GND) SMA21.GND@1(GND) SMA21.GND@2(GND) SMA21.GND@3(GND) SMA21.GND@4(GND) SMA30.GND@1(GND) SMA30.GND@2(GND) SMA30.GND@3(GND) SMA30.GND@4(GND) SMA31.GND@1(GND) SMA31.GND@2(GND) SMA31.GND@3(GND) SMA31.GND@4(GND) SMA40.GND@1(GND) SMA40.GND@2(GND) SMA40.GND@3(GND) SMA40.GND@4(GND) SMA41.GND@1(GND) SMA41.GND@2(GND) SMA41.GND@3(GND) SMA41.GND@4(GND) SWD.4 T1.2(E) U$1.1_GND U$1.10_GND U$1.12_GND USB.5 USB.M1(S1) USB.M2(S2)
GPS-1PPS: IC800.24(PA1) IC800.48(PB11) R703.1
GPS-RX: IC800.25(PA2) IC800.35(PB0) R701.1
GPS-TX: IC800.87(PD6) R700.1
GPS-VCC: C700.2 C701.2 R705.2 U$1.6_V_BCKP U$1.7_VCC_IO U$1.8_VCC U$1.9_RESET_N(9_V_RESET_N)
IC202: C216.2 IC205.3(CH1) R217.2
IC504IN: C514.1 C515.1 IC504.1(IN) R506.2
N$1: C505.1 IC500.3(+IN) R500.2 R501.1
N$2: IC100.1(OUT) R103.1 R104.1
N$3: C220.2 IC205.2(CH0) R218.2
N$4: C116.2 IC105.3(CH1) R117.2
N$5: IC106.4(-IN) R121.1
N$6: IC100.4(-IN) R102.1 R103.2
N$7: IC101.4(IN-) R111.2 R112.1
N$8: C120.2 IC105.2(CH0) R118.2
N$9: LED1.A R503.1
N$10: C813.2 IC800.13(PH1) Q2.2
N$11: C406.2 L401.2 L402.1
N$12: IC500.1(OUT) R502.2
N$13: IC105.1(VOUT) R119.1
N$14: C413.2 IC402.2(CH0) R414.2
N$15: C320.2 IC305.2(CH0) R318.2
N$16: IC205.1(VOUT) R219.1
N$17: C203.2 R201.1 R205.2 R206.1 R207.1 TR2.4(S2)
N$18: C207.2 C208.1 C209.1 L202.2 R208.2
N$19: C205.2 L200.2 L201.1
N$20: IC305.1(VOUT) R319.1
N$21: C306.2 L301.2 L302.1
N$22: C213.2 IC202.2(CH0) R214.2
N$23: C209.2 C210.1 R209.2
N$24: C210.2 C211.1 R213.1
N$25: C229.1 SMA20.SIG
N$26: C313.1 IC301.1(OUT) R312.2 R313.2
N$27: IC405.1(VOUT) R419.1
N$28: C211.2 IC201.3(IN+) R210.2
N$29: IC200.1(OUT) R203.1 R204.1
N$30: C308.2 IC302.3(CH1) R315.2
N$31: C204.2 L200.1 R206.2
N$32: C124.2 R120.2
N$33: IC201.4(IN-) R211.2 R212.1
N$34: IC200.4(-IN) R202.1 R203.2
N$35: IC600.14(RBIAS) R606.2
N$36: IC106.1(OUT) R120.1 R121.2
N$37: C213.1 IC201.1(OUT) R212.2 R213.2
N$38: C208.2 IC202.3(CH1) R215.2
N$39: C113.1 IC101.1(OUT) R112.2 R113.2
N$40: C420.2 IC405.2(CH0) R418.2
N$41: C124.1 SMA11.SIG
N$42: C307.2 C308.1 C309.1 L302.2 R308.2
N$43: C305.2 L300.2 L301.1
N$44: C404.2 L400.1 R406.2
N$45: C603.2 IC600.24(OSC2) Q1.1
N$46: C313.2 IC302.2(CH0) R314.2
N$47: C309.2 C310.1 R309.2
N$48: C310.2 C311.1 R313.1
N$49: C413.1 IC401.1(OUT) IC401.4(IN-) R413.2
N$50: C311.2 IC301.3(IN+) R310.2
N$51: C429.1 SMA40.SIG
N$52: C329.2 R304.2
N$53: IC301.4(IN-) R311.2 R312.1
N$54: C403.2 C430.2 R401.1 R405.1 R406.1 R407.1
N$55: C216.1 C217.1 IC202.1(VOUT)
N$56: C206.2 L201.2 L202.1
N$57: IC300.1(OUT) R303.1 R304.1
N$58: C224.2 R220.2
N$59: C405.2 L400.2 L401.1
N$60: C224.1 SMA21.SIG
N$61: C602.2 IC600.23(OSC1) Q1.2
N$62: IC206.1(OUT) R220.1 R221.2
N$63: C324.2 R320.2
N$64: C407.2 C408.1 C410.1 L402.2 R408.1
N$65: C410.2 C411.1 R413.1
N$66: IC406.1(OUT) R420.1 R421.2
N$67: C411.2 IC401.3(IN+) R410.2
N$68: C106.2 L101.2 L102.1
N$69: IC600.27(LEDA) R600.1
N$70: C408.2 IC402.3(CH1) R415.2
N$71: IC306.1(OUT) R320.1 R321.2
N$72: H-INPUT.1 R100.2 TR1.1
N$73: H-INPUT.2 R100.1 TR1.3(P2)
N$74: H-INPUT.3 R200.2 TR2.1
N$75: H-INPUT.6 R200.1 TR2.3(P2)
N$76: H-INPUT.7 R300.2 TR3.1
N$77: H-INPUT.8 R300.1 TR3.3(P2)
N$78: IC300.4(-IN) R302.1 R303.2
N$79: R600.2 RJ1.G+
N$80: C108.2 IC102.3(CH1) R115.2
N$81: IC400.1(OUT) R403.1 R404.1
N$82: IC600.26(LEDB) R601.1
N$83: C217.2 IC203.1(IN+) R216.2
N$84: C220.1 IC203.8(OUT)
N$85: C110.2 C111.1 R113.1
N$86: IC400.4(-IN) R402.1 R403.2
N$87: C117.2 IC103.1(IN+) R116.2
N$88: C303.2 R301.1 R305.2 R306.1 R307.1 TR3.4(S2)
N$89: C111.2 IC101.3(IN+) R110.2
N$90: C120.1 IC103.8(OUT)
N$91: C107.2 C108.1 C109.1 L102.2 R108.2
N$92: C105.2 L100.2 L101.1
N$93: C316.1 C317.1 IC302.1(VOUT)
N$94: C113.2 IC102.2(CH0) R114.2
N$95: C316.2 IC305.3(CH1) R317.2
N$96: C109.2 C110.1 R109.2
N$97: R601.2 RJ1.Y+
N$98: C116.1 C117.1 IC102.1(VOUT)
N$99: C317.2 IC303.1(IN+) R316.2
N$100: C320.1 IC303.8(OUT)
N$101: C605.2 IC600.1(VCAP)
N$102: C416.1 C417.1 IC402.1(VOUT)
N$103: C416.2 IC405.3(CH1) R417.2
N$104: C417.2 IC403.1(IN+) R416.2
N$105: C420.1 IC403.8(OUT)
N$106: C104.2 L100.1 R106.2
N$107: C424.2 R420.2
N$108: IC600.10(!RESET) R607.1
N$109: C424.1 SMA41.SIG
N$110: C600.2 C607.1 R602.2 R603.2 R608.2 R609.2 RJ1.P4
N$111: C304.2 L300.1 R306.2
N$112: IC600.17(TPOUT+) R603.1 RJ1.TD+
N$113: IC600.16(TPOUT-) R602.1 RJ1.TD-
N$114: C129.1 SMA10.SIG
N$115: C702.1 C703.1 R702.2 R704.2 U$1.14_VCC_RF
N$116: IC600.12(TPIN-) R604.2 RJ1.RD-
N$117: IC600.13(TPIN+) R605.2 RJ1.RD+
N$118: C601.2 R604.1 R605.1
N$119: BUZZER.+ R800.1 T1.3(C)
N$120: R801.1 R802.2 T1.1(B)
N$121: C814.2 IC800.12(PH0) Q2.1
N$122: C502.1 C503.1 IC501.1(IN) IC501.3(EN) R508.2 R511.2
N$123: LED5.A R806.1
N$124: IC206.4(-IN) R221.1
N$125: C516.1 C517.1 IC505.1(IN) R507.2
N$126: IC800.55(PD8) J1.1 R821.2
N$127: IC800.59(PD12) J0.1 R822.2
N$128: IC306.4(-IN) R321.1
N$129: LED4.A R808.1
N$130: LED3.A R812.1
N$131: C329.1 SMA30.SIG
N$132: C429.2 R404.2
N$133: C229.2 R204.2
N$135: IC800.26(PA3) R823.2 R824.1
N$136: IC406.4(-IN) R421.1
N$137: C324.1 SMA31.SIG
N$138: LED2.A R816.1
N$139: IC800.77(PA15) R812.2 R813.2
N$140: IC800.3(PE4) R816.2 R817.2
N$141: R702.1 U$1.15_V_ANT/RESERVED(15_RES/V_ANT)
N$146: C129.2 R104.2
N$147: GPS-IN.SIG U$1.11_RF_IN
N$148: C807.2 C809.2 IC800.22(VDDA) R804.1 R826.1 R831.1
N$149: IC800.81(PD0) R808.2 R809.2
N$150: C810.1 IC800.49(VCAP_1)
N$151: LED1B.A R504.1
N$152: IC800.83(PD2) R806.2 R807.2
N$153: C811.1 IC800.73(VCAP_2)
N$154: BOOT0.3(P) BOOT0.4(P1) IC800.94(BOOT0) R805.2
N$155: LED7.A R814.1
N$156: LED6.A R810.1
N$157: IC800.84(PD3) R814.2 R815.2
N$158: IC800.85(PD4) R810.2 R811.2
N$159: R819.2 SERIAL.3
N$160: R820.2 SERIAL.4
N$161: IC800.68(PA9) J3.2
N$162: LED2B.A R817.1
N$163: LED3B.A R813.1
N$164: LED6B.A R811.1
N$165: LED7B.A R815.1
N$166: LED4B.A R809.1
N$167: LED5B.A R807.1
N$197: C506.1 C507.1 IC503.1(IN) IC503.3(EN) R509.2 R510.2
N$199: C508.1 C509.1 IC502.1(IN) R505.2
N$200: F600.2 R609.1
N$201: C608.1 R608.1
N$202: F800.1 R826.2
N$203: C818.1 R831.2
N$204: F502.2 R509.1
N$205: C521.2 R510.1
N$206: C522.2 R511.1
N$207: F501.2 R508.1
N$208: C430.1 E-INPUT.1 L403.2
N$209: F700.2 R705.1
N$210: C704.1 R704.1
N$211: IC800.54(PB15) R828.1
N$212: IC800.52(PB13) R829.1
N$213: IC800.51(PB12) R830.1
RESET: C812.1 IC800.14(NRST) R803.1 RESET.1(S) RESET.2(S1)
RX: R701.2 U$1.3_RXD
S2: IC402.8(SO) IC405.7(SI)
S3: IC302.7(SI) IC405.8(SO)
S4: IC302.8(SO) IC305.7(SI)
S5: IC202.7(SI) IC305.8(SO)
S6: IC202.8(SO) IC205.7(SI)
S7: IC102.7(SI) IC205.8(SO)
S8: IC102.8(SO) IC105.7(SI)
SCK: IC102.9(SCK) IC105.9(SCK) IC202.9(SCK) IC205.9(SCK) IC302.9(SCK) IC305.9(SCK) IC402.9(SCK) IC405.9(SCK) IC800.89(PB3)
SERIAL-RX: IC800.78(PC10) R820.1
SERIAL-TX: IC800.79(PC11) R819.1
SI: IC402.7(SI) IC800.91(PB5)
SWCLK: IC800.76(PA14) SWD.3
SWDIO: IC800.72(PA13) SWD.2
T_OUT_1: IC100.3(+IN) R101.2
T_OUT_2: IC300.3(+IN) R301.2
T_OUT_3: IC400.3(+IN) R401.2
T_OUT_5: IC200.3(+IN) R201.2
T_OUT_7: C323.1 IC306.3(+IN) L304.2 R319.2
TP: C103.1 C203.1 C303.1 C403.1 IC800.29(PA4) R107.2 R207.2 R307.2 R407.2
TX: R700.2 U$1.2_TXD
USBD+: IC800.71(PA12) R825.1 USB.3
USBD-: IC800.70(PA11) USB.2
USBID: IC800.69(PA10) USB.4
USBV: F500.2 POWER.1
USBV0: POWER.2 USB.1
V+: BUZZER.- C500.1 C501.1 C511.1 C512.1 C519.+ C520.+ F500.1 F501.1 F502.1 J3.1 R503.2 R504.2 R505.1 R506.1 R507.1 R800.2 R824.2 SERIAL.1 SWD.5
VDD: C102.2 C112.2 C115.2 C122.2 C125.2 C202.2 C212.2 C215.2 C222.2 C225.2 C302.2 C312.2 C315.2 C322.2 C325.2 C402.2 C412.2 C415.2 C422.2 C425.2 C504.1 IC100.5(V+) IC101.5(+VS) IC102.10(VDD) IC105.10(VDD) IC106.5(V+) IC200.5(V+) IC201.5(+VS) IC202.10(VDD) IC205.10(VDD) IC206.5(V+) IC300.5(V+) IC301.5(+VS) IC302.10(VDD) IC305.10(VDD) IC306.5(V+) IC400.5(V+) IC401.5(+VS) IC402.10(VDD) IC405.10(VDD) IC406.5(V+) IC500.5(V+) IC501.5(OUT)
VREF: C806.1 C808.1 IC800.21(VREF+) R500.1 R804.2
Unconnected: IC104.1(NC) IC105.8(SO) IC204.1(NC) IC304.1(NC) IC404.1(NC) IC600.3(CLKOUT) IC600.5(NC*) IC800.1(PE2) IC800.4(PE5) IC800.6(VBAT) IC800.7(PC13) IC800.9(PC15) IC800.15(PC0) IC800.17(PC2) IC800.18(PC3) IC800.23(PA0) IC800.31(PA6) IC800.32(PA7) IC800.38(PE7) IC800.39(PE8) IC800.41(PE10) IC800.42(PE11) IC800.43(PE12) IC800.44(PE13) IC800.45(PE14) IC800.46(PE15) IC800.47(PB10) IC800.56(PD9) IC800.60(PD13) IC800.61(PD14) IC800.62(PD15) IC800.63(PC6) IC800.64(PC7) IC800.65(PC8) IC800.67(PA8) IC800.80(PC12) IC800.86(PD5) IC800.88(PD7) IC800.90(PB4) IC800.92(PB6) IC800.93(PB7) IC800.95(PB8) IC800.97(PE0) IC800.98(PE1) RJ1.NC RJ1.P5 U$1.5_EXTINT U$1.13_LNA_EN(13_LNA_EN/RES) U$1.16_SDA U$1.17_SCL U$1.18_SAFEBOOT_N

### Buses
CLK1I,CLK2I,CLK3I,CLK4I
CLK1,CLK2,CLK3,CLK4
SCK,SI,CS
ENC28J60-CS,ENC28J60-INT,ENC28J60-SCK,ENC28J60-SI,ENC28J60-SO
GPS-1PPS,GPS-RX,GPS-TX
AMP-CH1,AMP-CH2,AMP-CH3,AMP-CH4

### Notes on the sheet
- 20-Feb-2018

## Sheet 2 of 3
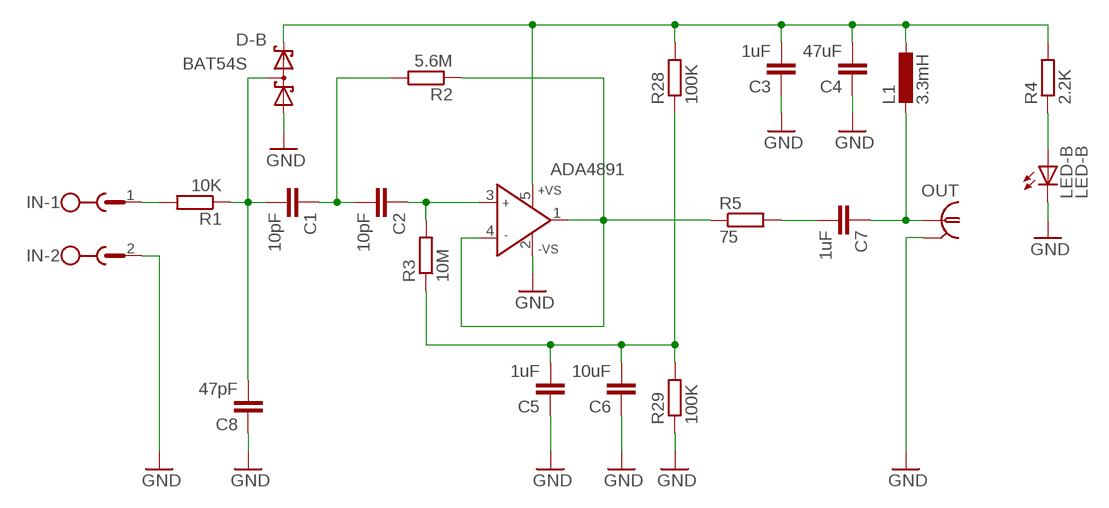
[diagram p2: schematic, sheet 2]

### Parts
C1  10pF  C-EUC0603  [C0603]
C2  10pF  C-EUC0603  [C0603]
C3  1uF  C-EUC0603  [C0603]
C4  47uF  C-EUC1210  [C1210]
C5  1uF  C-EUC0603  [C0603]
C6  10uF  C-EUC0805  [C0805]
C7  1uF  C-EUC0603  [C0603]
C8  47pF  C-EUC0603  [C0603]
D-B  BAT54S  [SOT23]
IC1  ADA4891  AD8614RJ  [SOT23-5]
IN  MSTBV2  [MSTBV2]
L1  3.3mH  L-EU6000-XXX-RC  [6000-XXXX-RC]
LED-B  LED-B  LEDCHIP-LED0805  [CHIP-LED0805]
OUT  R141426  [R141426]
R1  10K  R-EU_R0603  [R0603]
R2  5.6M  R-EU_R0603  [R0603]
R3  10M  R-EU_R0603  [R0603]
R4  2.2K  R-EU_R0603  [R0603]
R5  75  R-EU_R0603  [R0603]
R28  100K  R-EU_R0603  [R0603]
R29  100K  R-EU_R0603  [R0603]

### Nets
ADA4891: IC1.1(OUT) IC1.4(IN-) R2.1 R5.1
E-ANTENNE: IN.1 R1.2
GND-B: C3.1 C4.1 C5.1 C6.1 C8.1 D-B.1(A1) IC1.2(-VS) IN.2 LED-B.C OUT.2(GND) R29.1 ; supply symbol labelled GND
N$142: C7.1 L1.2 OUT.1
N$143: C7.2 R5.2
N$144: C2.1 IC1.3(IN+) R3.2
N$145: C1.1 C2.2 R2.2
N$168: C1.2 C8.2 D-B.3(C1A2) R1.1
N$169: LED-B.A R4.1
N$170: C5.2 C6.2 R3.1 R28.1 R29.2
V+B: C3.2 C4.2 D-B.2(C2) IC1.5(+VS) L1.1 R4.2 R28.2

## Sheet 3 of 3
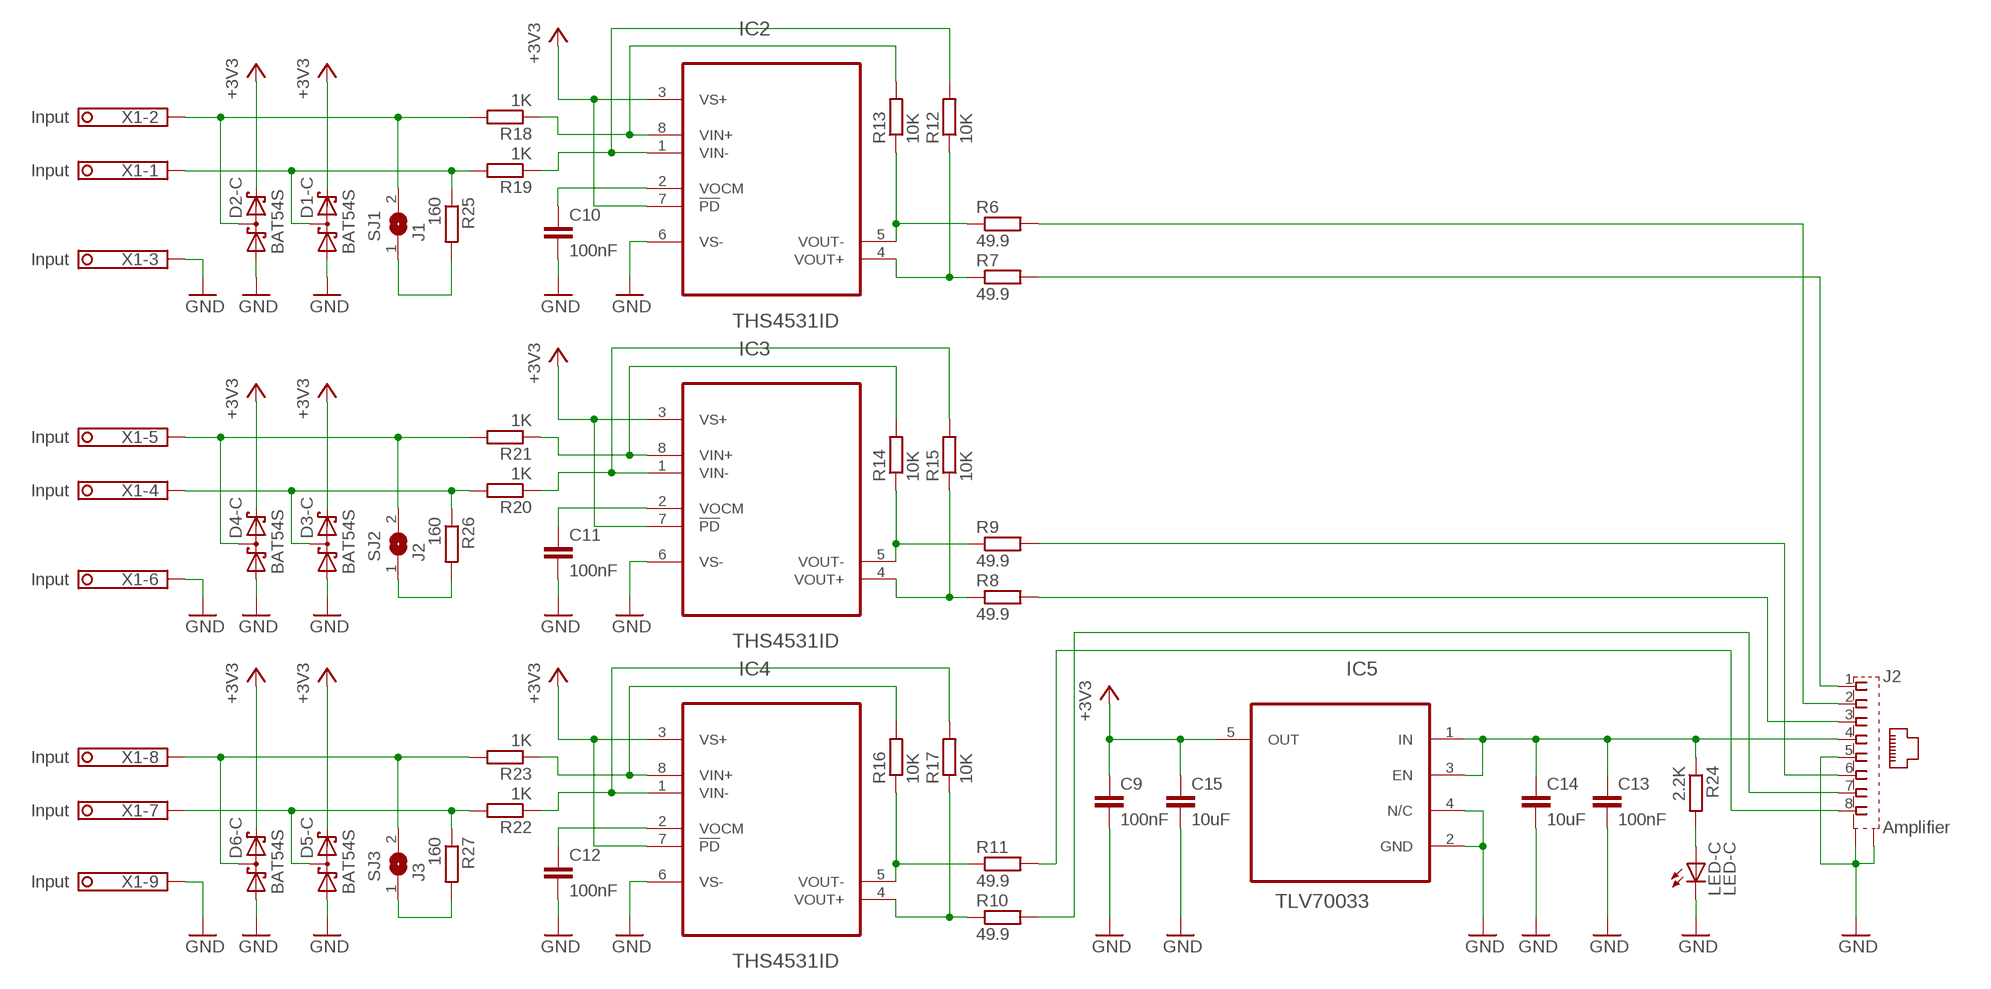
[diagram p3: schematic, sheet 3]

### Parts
C9  100nF  C-EUC0603  [C0603]
C10  100nF  C-EUC0603  [C0603]
C11  100nF  C-EUC0603  [C0603]
C12  100nF  C-EUC0603  [C0603]
C13  100nF  C-EUC0603  [C0603]
C14  10uF  C-EUC0805  [C0805]
C15  10uF  C-EUC0805  [C0805]
D1-C  BAT54S  [SOT23]
D2-C  BAT54S  [SOT23]
D3-C  BAT54S  [SOT23]
D4-C  BAT54S  [SOT23]
D5-C  BAT54S  [SOT23]
D6-C  BAT54S  [SOT23]
IC2  THS4531ID  [SOIC127P600X175-8N]
IC3  THS4531ID  [SOIC127P600X175-8N]
IC4  THS4531ID  [SOIC127P600X175-8N]
IC5  TLV70033  TLV70033DDCT  [SOT95P280X110-5N]
J2  Amplifier  556591-1  [556591-1]
LED-C  LED-C  LEDCHIP-LED0805  [CHIP-LED0805]
R6  49.9  R-EU_R0603  [R0603]
R7  49.9  R-EU_R0603  [R0603]
R8  49.9  R-EU_R0603  [R0603]
R9  49.9  R-EU_R0603  [R0603]
R10  49.9  R-EU_R0603  [R0603]
R11  49.9  R-EU_R0603  [R0603]
R12  10K  R-EU_R0603  [R0603]
R13  10K  R-EU_R0603  [R0603]
R14  10K  R-EU_R0603  [R0603]
R15  10K  R-EU_R0603  [R0603]
R16  10K  R-EU_R0603  [R0603]
R17  10K  R-EU_R0603  [R0603]
R18  1K  R-EU_R0603  [R0603]
R19  1K  R-EU_R0603  [R0603]
R20  1K  R-EU_R0603  [R0603]
R21  1K  R-EU_R0603  [R0603]
R22  1K  R-EU_R0603  [R0603]
R23  1K  R-EU_R0603  [R0603]
R24  2.2K  R-EU_R0603  [R0603]
R25  160  R-EU_R0603  [R0603]
R26  160  R-EU_R0603  [R0603]
R27  160  R-EU_R0603  [R0603]
SJ1  J1  SJ  [SJ]
SJ2  J2  SJ  [SJ]
SJ3  J3  SJ  [SJ]
X1  Input  1751316  [1751316]

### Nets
+3V3-C: C9.1 C15.1 D1-C.2(C2) D2-C.2(C2) D3-C.2(C2) D4-C.2(C2) D5-C.2(C2) D6-C.2(C2) IC2.3(VS+) IC2.7(!PD) IC3.3(VS+) IC3.7(!PD) IC4.3(VS+) IC4.7(!PD) IC5.5(OUT) ; supply symbol labelled +3V3
A1: IC4.4(VOUT+) R10.1 R17.1
A2: IC3.4(VOUT+) R8.1 R15.1
A3: IC2.4(VOUT+) R7.1 R12.1
GND-C: C9.2 C10.2 C11.2 C12.2 C13.2 C14.2 C15.2 D1-C.1(A1) D2-C.1(A1) D3-C.1(A1) D4-C.1(A1) D5-C.1(A1) D6-C.1(A1) IC2.6(VS-) IC3.6(VS-) IC4.6(VS-) IC5.2(GND) IC5.4(N/C) J2.5 J2.G1(S1) J2.G2(S2) LED-C.C X1.3 X1.6 X1.9 ; supply symbol labelled GND
I1A: D2-C.3(C1A2) R18.2 SJ1.2 X1.2
I1B: D1-C.3(C1A2) R19.2 R25.1 X1.1
I2A: D4-C.3(C1A2) R21.2 SJ2.2 X1.5
I2B: D3-C.3(C1A2) R20.2 R26.1 X1.4
I3A: D6-C.3(C1A2) R23.2 SJ3.2 X1.8
I3B: D5-C.3(C1A2) R22.2 R27.1 X1.7
N$171: IC3.5(VOUT-) R9.1 R14.1
N$172: IC4.5(VOUT-) R11.1 R16.1
N$173: IC2.5(VOUT-) R6.1 R13.1
N$174: J2.1 R7.2
N$175: J2.2 R6.2
N$176: J2.3 R8.2
N$177: J2.6 R9.2
N$178: J2.7 R10.2
N$179: J2.8 R11.2
N$180: IC2.1(VIN-) R12.2 R19.1
N$181: IC2.8(VIN+) R13.2 R18.1
N$182: IC3.8(VIN+) R14.2 R21.1
N$183: IC3.1(VIN-) R15.2 R20.1
N$184: IC4.8(VIN+) R16.2 R23.1
N$185: IC4.1(VIN-) R17.2 R22.1
N$186: C10.1 IC2.2(VOCM)
N$187: C11.1 IC3.2(VOCM)
N$188: C12.1 IC4.2(VOCM)
N$189: C13.1 C14.1 IC5.1(IN) IC5.3(EN) J2.4 R24.1
N$190: LED-C.A R24.2
N$191: R27.2 SJ3.1
N$192: R26.2 SJ2.1
N$193: R25.2 SJ1.1

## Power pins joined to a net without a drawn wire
GND: E-INPUT.3(GND) E-INPUT.4(GND) E-INPUT.5(GND)
GND-B: OUT.3(GND) OUT.4(GND) OUT.5(GND)

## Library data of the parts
BOOT0 BOOT1 RESET = switch-omron:10-XX: OMRON SWITCH; MPN: B3F-1000; OC_FARNELL: 176432; OC_NEWARK: 36M3542
BUZZER = buzzer:F/CM12P: BUZZER; OC_FARNELL: unknown; OC_NEWARK: unknown
C1-C15 C100-C125 C127-C129 C200-C225 C227-C229 C300-C325 C327-C329 C400-C408 C410-C425 C427-C430 C500-C518 C521 C522 C600-C608 C700-C704 C800-C818 = rcl:C-EU: CAPACITOR, European symbol
C519 C520 = rcl:CPOL-US: POLARIZED CAPACITOR, American symbol; SPICEPREFIX: C
D1-C D2-C D3-C D4-C D5-C D6-C D-B = diode:BAT54S: Schottky Diodes Pin connection corrected 2011-05-04 Source: Fairchild .. BAT54.pdf
E-INPUT OUT = con-coax:R141426: BNC COAX CONNECTOR Radiall 50/75 Ohm Spoerle; MF: FARNELL; MPN: R141426161; OC_FARNELL: 4195115; OC_NEWARK: 14J7919
F500-F502 F600 F700 F800 L100-L102 L104 L200-L202 L204 L300-L302 L304 L400-L402 L404 R1-R29 R100-R121 R200-R221 R300-R321 R401-R408 R410 R413-R421 R500-R511 R600-R611 R700-R705 R800-R826 R828-R831 = rcl:R-EU_: RESISTOR, European symbol
GPS-IN SMA10 SMA11 SMA20 SMA21 SMA30 SMA31 SMA40 SMA41 = connectors:XS-4S: Shielded connector, 4 shield pins - LEMO 00 - SMA
H-INPUT J2 = con-amp:556591-1: AMP connector
IC1 IC101 IC201 IC301 IC401 = analog-devices:AD8614: Single and Quad 18 V Operational Amplifiers Source: http://www.analog.com/static/imported-files/data_sheets/AD8614_8644.pdf; MF: ALTERA CORPORATION; MPN: AD8614ARTZ-REEL7; OC_FARNELL: 1464998; OC_NEWARK: 88H0303
IC2-IC4 = THS4531ID:THS4531ID: Ultra Low Power, Rail-to-Rail Output, Fully-Differential Amplifier,SOIC-8; MPN: THS4531ID; OC_FARNELL: 2115228; OC_NEWARK: 05W5826; PACKAGE: SOIC- 8; SUPPLIER: TEXAS INSTRUMENTS
IC5 IC501 IC503 = TLV70033:TLV70033DDCT: 200-mA, Low-IQ, Low-Dropout Regulator for Portable Devices; MPN: TLV70033DDCT; OC_FARNELL: 1778230; OC_NEWARK: 50R4446; PACKAGE: TSOT-23-5; SUPPLIER: Texas Instruments
IC100 IC106 IC200 IC206 IC300 IC306 IC400 IC406 IC500 = linear:OPA*-SOT23: Single Operational Amplifier Low Power, Single-Supply, Rail-To-Rail Operational Amplifier Source: http://focus.ti.com/lit/ds/symlink/opa2345.pdf
IC102 IC105 IC202 IC205 IC302 IC305 IC402 IC405 = MCP6S93:MCP6S93-E/UN: AMP PROGRAMMABLE GAIN 2 CH; MPN: MCP6S93-E/UN; OC_FARNELL: 9190520; OC_NEWARK: 92K6752; PACKAGE: 10 MSOP; SUPPLIER: Microchip
IC103 IC203 IC303 IC403 = Blitzortung:LTC1569-7
IC104 IC204 IC304 IC404 = 74HC1G04DTT1G:MC74HC1G04DTT1G: Single Inverter; MPN: MC74HC1G04DTT1G; OC_FARNELL: 1706041; OC_NEWARK: 95K5518; PACKAGE: SOT-23-5; SUPPLIER: ON SEMICONDUCTOR
IC502 IC504 IC505 = LM3940IMP-3.3:LM3940IMP-3.3: Low Dropout Regulator; MPN: LM3940IMP-33; OC_FARNELL: 9779280; OC_NEWARK: 7B6637; PACKAGE: SOT-223-4; SUPPLIER: TEXAS INSTRUMENTS
IC600 = microchip-6:ENC28J60: Stand-Alone Ethernet Controller with SPI Interface Source: http://ww1.microchip.com/downloads/en/DeviceDoc/39662c.pdf
IC800 = stm32f:STM32F40X: Features • Core: ARM 32-bit Cortex™-M4 CPU with FPU, Adaptive real-time accelerator (ART Accelerator™) allowing 0-wait state execution from Flash memory, frequency up to 168 MHz, memory protection unit, 210 DMIPS/ 1.25 DMIPS/MHz (Dhrystone 2.1), and DSP instructions • Memories – Up to 1 Mbyte of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
IN = con-phoenix-508:MSTBV2: PHOENIX; MPN: MSTBV 2,5/2-GF-5.08; OC_FARNELL: 1792792; OC_NEWARK: 69R9845
J0 J1 J3 SJ1-SJ3 = jumper:SJ: SMD solder JUMPER
L1 L403 = rcl:L-EU: INDUCTOR, European symbol; SPICEPREFIX: L
LED1 LED1B LED2 LED2B LED3 LED3B LED4 LED4B LED5 LED5B LED6 LED6B LED7 LED7B LED-B LED-C = led:LED: LED
POWER = pinhead:PINHD-1X2: PIN HEADER
Q1 Q2 = crystal:CRYSTAL: CRYSTAL; OC_FARNELL: 1666969; OC_NEWARK: unknown
RJ1 = HanRun:HR911105A
SERIAL SWD = connectors:X05: Connector 5 pins
T1 = transistor-npn:BC847*: NPN Transistor
TR1-TR3 = trafo-murata:78601
U$1 = ublox:MAX-M8: u-blox MAX GNSS module
USB = con-cypressindustries:MINI-USB_SHIELD5P2-: MINI USB-B R/A DIP 5pol. Source: www.cypressindustries.com; OC_FARNELL: unknown; OC_NEWARK: unknown
X1 = con-phoenix-350:1751316: MKDS 1/ 9-3,5 Printklemme Nennstrom: 10 A Bemessungsspannung: 160 V Raster: 3,5 mm Polzahl: 9 Montageart: Löten Anschlussart: Schraubanschluss Anschlussrichtung vom Leiter zur Platine: 0° Source: http://eshop.phoenixcontact.com .. 1751316.pdf; OC_FARNELL: unknown; OC_NEWARK: unknown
